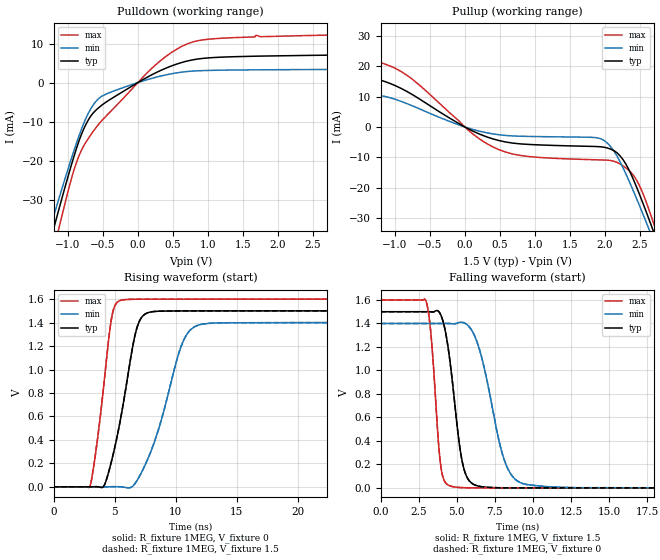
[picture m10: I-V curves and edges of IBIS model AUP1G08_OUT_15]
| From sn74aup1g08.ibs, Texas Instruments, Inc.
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[Model]   AUP1G08_OUT_15
Model_type  Output
Vref =   0
Rref =   1E6
Cref =   30p
Vmeas =   0.75
| variable   typ   min   max
C_comp   2.94pF   2.15pF   4.08pF
| C_pullup   3.16pF   2.15pF   4.08pF
| C_pulldown   2.72pF   2.30pF   3.22pF
[Temperature Range]   40   100   -40
| Ambient temperature   25   85   -40
[Voltage range]   1.5   1.4   1.6
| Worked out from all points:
|   slope of the pulldown table from 0 to 0.225 V, typ, clamps not added: 101 ohm
|   slope of the pullup table from 0 to 0.225 V, typ, clamps not added: 90.4 ohm
|   rising waveform, R_fixture 1MEG, V_fixture 0: 20-80 % time 1.56ns typ, 2.32ns min, 1.05ns max; typ from 0 V to 1.5 V
|   falling waveform, R_fixture 1MEG, V_fixture 1.5: 20-80 % time 828ps typ, 1.4ns min, 515ps max; typ from 1.5 V to 0 V
|   rising waveform, R_fixture 1MEG, V_fixture 1.5: 20-80 % time 1.56ns typ, 2.32ns min, 1.05ns max; typ from 0 V to 1.5 V
|   falling waveform, R_fixture 1MEG, V_fixture 0: 20-80 % time 828ps typ, 1.4ns min, 515ps max; typ from 1.5 V to 0 V
[Pulldown]
| AUP1G08_OUT_15
|   Voltage   I(typ)   I(min)   I(max)
-3.6V     -206.2mA   -188.5mA   -228mA
-1.265V   -41.61mA   -37.97mA   -47.66mA
-1.21V    -37.92mA   -34.65mA   -43.5mA
-1.11V    -31.31mA   -28.69mA   -36.01mA
-945mV    -20.85mA   -19.22mA   -24.38mA
-855mV    -15.71mA   -14.4mA    -19.43mA
-720mV    -9.974mA   -8.304mA   -14.65mA
-570mV    -6.595mA   -4.271mA   -10.91mA
260mV     2.544mA    1.373mA    4.642mA
810mV     5.906mA    2.979mA    10.53mA
1.69V     6.763mA    3.269mA    12.06mA
7.2V      7.827mA    3.609mA    13.77mA
[Pullup]
| AUP1G08_OUT_15
|   Voltage   I(typ)   I(min)   I(max)
-3.6V     29.66mA    17.92mA    40.73mA
-2.925V   22.54mA    13.62mA    31.92mA
-2.13V    15.77mA    9.482mA    23.18mA
-1.025V   13.91mA    9.316mA    19.64mA
130mV     -1.525mA   -910.1uA   -2.565mA
590mV     -4.979mA   -2.819mA   -8.32mA
1.925V    -6.506mA   -3.765mA   -10.85mA
2.175V    -8.514mA   -9.578mA   -11.67mA
2.395V    -16.55mA   -20.33mA   -15.49mA
2.615V    -29.33mA   -32.65mA   -26.16mA
2.72V     -35.91mA   -38.77mA   -33.21mA
7.2V      -352.8mA   -330.6mA   -379.7mA
[Ramp]
| AUP1G08_OUT_15
| variable   typ   min   max
dV/dt_r   0.90/1.57E-09   0.85/2.34E-09   0.96/1.06E-09
dV/dt_f   0.91/8.36E-10   0.85/1.41E-09   0.96/5.20E-10
R_load = 1MEG
[Rising Waveform]
| AUP1G08_OUT_15
R_fixture =   1MEG
C_fixture =   0
L_fixture =   0
V_fixture =   0
V_fixture_min = 0
V_fixture_max = 0
|   Time   V(typ)   V(min)   V(max)
0s        19.89nV    117.7nV    1.066nV
2.975ns   -77.63uV   -208.9nV   10.5mV
4.06ns    772.5uV    -96.49uV   832mV
4.695ns   204.7mV    739.9uV    1.414V
5.41ns    545mV      393.4uV    1.587V
6.565ns   1.25V      15.61mV    1.599V
7.175ns   1.441V     120.2mV    1.599V
10.46ns   1.499V     1.205V     1.6V
11.75ns   1.5V       1.374V     1.6V
40ns      1.5V       1.4V       1.6V
[Falling Waveform]
| AUP1G08_OUT_15
R_fixture =   1MEG
C_fixture =   0
L_fixture =   0
V_fixture =   1.5
V_fixture_min = 1.4
V_fixture_max = 1.6
|   Time   V(typ)   V(min)   V(max)
0s        1.5V       1.4V       1.6V
2.975ns   1.5V       1.4V       1.591V
3.31ns    1.499V     1.4V       1.294V
3.94ns    1.474V     1.4V       191.2mV
4.6ns     1.025V     1.399V     14.74mV
5.23ns    314.8mV    1.41V      2.694mV
5.72ns    77.9mV     1.385V     749.2uV
8.125ns   676.2uV    234.1mV    84.42uV
9.335ns   204.7uV    36.66mV    81.3uV
40ns      139.6uV    237.8uV    80.77uV
[Rising Waveform]
| AUP1G08_OUT_15
R_fixture =   1MEG
C_fixture =   0
L_fixture =   0
V_fixture =   1.5
V_fixture_min = 1.4
V_fixture_max = 1.6
|   Time   V(typ)   V(min)   V(max)
0s        139.7uV    237.8uV    80.77uV
2.975ns   62.01uV    237.4uV    10.61mV
4.06ns    958.7uV    141.2uV    832.8mV
4.69ns    203.2mV    967.9uV    1.411V
5.41ns    546mV      629uV      1.588V
6.565ns   1.25V      16.05mV    1.599V
7.175ns   1.442V     121mV      1.599V
10.45ns   1.499V     1.205V     1.6V
11.74ns   1.5V       1.375V     1.6V
40ns      1.5V       1.4V       1.6V
[Falling Waveform]
| AUP1G08_OUT_15
R_fixture =   1MEG
C_fixture =   0
L_fixture =   0
V_fixture =   0
V_fixture_min = 0
V_fixture_max = 0
|   Time   V(typ)   V(min)   V(max)
0s        1.5V       1.4V       1.6V
2.975ns   1.5V       1.4V       1.591V
3.31ns    1.499V     1.4V       1.294V
3.94ns    1.474V     1.4V       190.9mV
4.6ns     1.024V     1.399V     14.64mV
5.23ns    314.3mV    1.41V      2.609mV
5.72ns    77.64mV    1.384V     667uV
8.125ns   532.7uV    233.5mV    3.621uV
9.335ns   64.42uV    36.36mV    525.3nV
40ns      -15.64nV   83.91nV    -4.491nV
